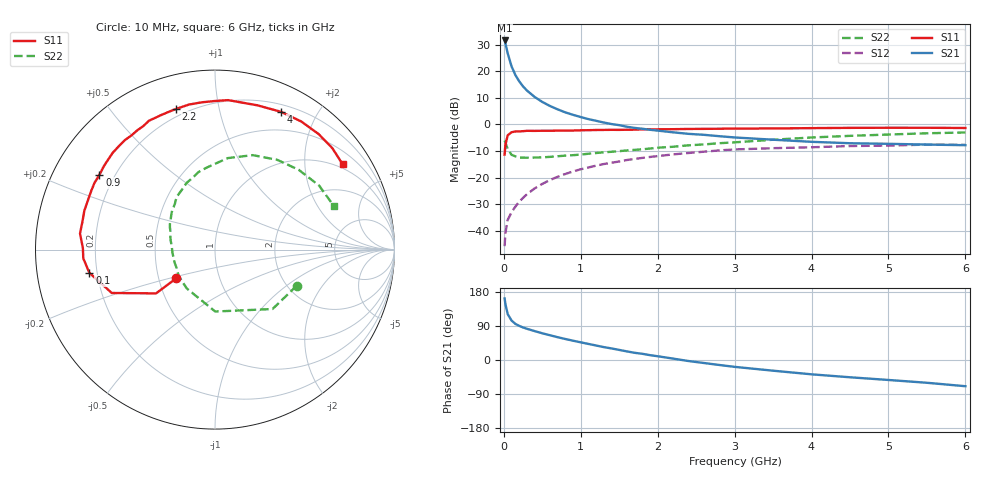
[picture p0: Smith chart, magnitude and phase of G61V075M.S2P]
! SIEMENS Small Signal Semiconductors
! BFG193
! Si NPN RF Bipolar Junction Transistor in SOT223
! VCE = 1 V  IC = 75 mA
! Common Emitter S-Parameters:  August  1996
# GHz  S  MA  R  50
!  f  S11  S21  S12  S22
! GHz  MAG  ANG  MAG  ANG  MAG  ANG  MAG  ANG
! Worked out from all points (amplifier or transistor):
!   36 points, 10 MHz to 6 GHz, reference 50 ohm
!   highest |S21| = 31.6 dB at 10 MHz (marker M1)
!   |S21| within 3 dB of that: start of sweep to 35.47 MHz
!   unconditionally stable (mu >= 1): start of sweep to 28.26 MHz; 104.4 MHz to end of sweep
!   at 250 MHz: K = 1.21, MAG = 18.2 dB, |S12| = -27.6 dB
!   at 1.4 GHz: K = 1.21, MAG = 4.5 dB, |S12| = -14.4 dB
!   at 6 GHz: K = 1.09, MAG = -1.8 dB, |S12| = -7.7 dB
!   S11 on the Smith chart (normalised r, x): 10 MHz: 0.62, -0.21; 100 MHz: 0.17, -0.09; 900 MHz: 0.14, +0.29; 2.2 GHz: 0.16, +0.75; 4 GHz: 0.28, +1.55; 6 GHz: 0.87, +3.08
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0.01  0.2696 -143.5  38.05 162.5  0.0051 67.9  0.4981 -23.8
0.02  0.4092 -143.4  33.72 148.1  0.009 62.3  0.4609 -45.9
0.05  0.6238 -157.2  21.81 121.1  0.0159 53.5  0.345 -89.8
0.1  0.7117 -169.5  12.41 104.2  0.0222 56.5  0.2675 -126.0
0.15  0.7355 -176.2  8.498 95.3  0.0283 59.2  0.2503 -144.1
0.2  0.7361 179.4  6.471 90.1  0.0351 62.1  0.2372 -153.9
0.25  0.7462 176.1  5.181 85.8  0.0415 64.1  0.2366 -162.5
0.3  0.7574 173.2  4.345 82.4  0.0484 65.1  0.2358 -167.2
0.4  0.7547 168.2  3.292 76.3  0.0623 65.6  0.2377 -175.8
0.5  0.7595 163.5  2.647 70.5  0.0759 64.1  0.24 177.8
0.6  0.7593 159.1  2.221 65.3  0.0898 63.1  0.2447 173.0
0.7  0.7631 154.7  1.919 60.1  0.1032 61.3  0.2513 168.9
0.9  0.7667 147.1  1.514 50.9  0.1302 56.8  0.2636 160.2
1.1  0.7781 140.1  1.257 42.4  0.1547 52.6  0.2803 153.7
1.6  0.7931 123.1  0.903 22.7  0.2135 39.7  0.3236 137.4
2.2  0.8131 105.6  0.709 3.7  0.2725 24.2  0.3796 119.4
2.8  0.8284 89.7  0.6 -13.1  0.3239 8.9  0.4425 101.8
3.5  0.8379 73.6  0.515 -28.2  0.3569 -9.6  0.5146 82.1
4  0.8512 64.4  0.47 -37.8  0.3712 -19.2  0.5669 68.2
4.5  0.8605 56.0  0.442 -45.6  0.3915 -29.1  0.6088 55.2
5.5  0.8642 40.9  0.417 -60.1  0.4167 -51.0  0.6809 31.6
6  0.8556 33.7  0.406 -69.2  0.4123 -63.5  0.7046 20.4
